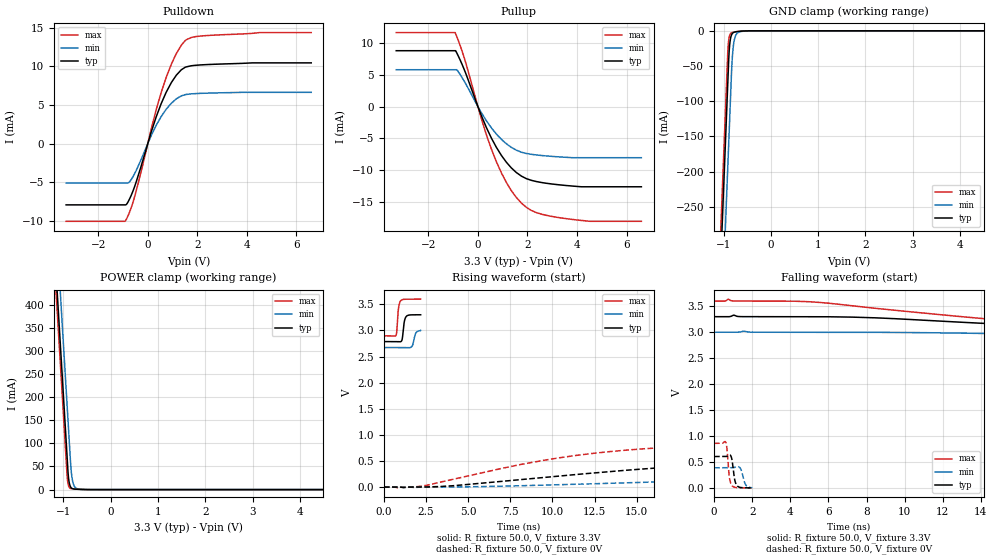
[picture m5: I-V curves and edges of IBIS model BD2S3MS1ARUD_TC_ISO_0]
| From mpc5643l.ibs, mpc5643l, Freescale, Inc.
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| *** New cell (Generated with 5.14beta1 (Sep 20 2010 13:23:23))
[Model]   BD2S3MS1ARUD_TC_ISO_0
Model_type I/O
Polarity   Non-Inverting
Enable   Active-Low
| CAP_THRESHOLD on pad pad is "CMOS" :
| Rising=10.0% of VDDE1   Falling=90.0% of VDDE1
| C_comp min and max val. don't necessarily correlate with the min and max pvt
| but are the smallest and greatest pad capacitance found.
| var   typ   min   max
C_comp   1.37510pF  1.31599pF  1.44239pF
Vinl = 1.05V | Dummy value overriden by next lines
Vinh = 2.34V | Dummy value overriden by next lines
Vmeas = 1.65V   | Reference voltage for timing measurements
Cref  = 25.0pF   | Timing specification test load capacitance value
Rref  = 1.0MOhm   | Timing specification test load resistance value
Vref  = 1.65V   | Timing specification test load voltage
[Model Spec]
| TIME_THRESHOLD on pin ipp_ind is "CORE" :
| Rising=40.0% of VDD   Falling=60.0% of VDD
Vinl 1.30950V 1.19650V 1.40650V
Vinh 1.89650V 1.72150V 2.04550V
| variable   typ   min   max
[Temperature Range] 25.0 150.0 -40.0
| variable   typ   min   max
[Voltage Range] 3.3V 3.0V 3.6V
| variable   typ   min   max
[POWER Clamp Reference] 3.3V 3.0V 3.6V
| variable   typ   min   max
[GND Clamp Reference] 0V 0V 0V
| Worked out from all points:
|   slope of the pulldown table from 0 to 0.495 V, typ, clamps not added: 104 ohm
|   slope of the pullup table from 0 to 0.495 V, typ, clamps not added: 108 ohm
|   GND clamp passes 1 mA (typ) near -0.70 V on its own axis
|   POWER clamp passes 1 mA (typ) near -0.74 V on its own axis
|   rising waveform, R_fixture 50.0, V_fixture 3.3V: 20-80 % time 118ps typ, 147ps min, 106ps max; typ from 2.79 V to 3.3 V
|   falling waveform, R_fixture 50.0, V_fixture 3.3V: 20-80 % time 19.3ns typ, 30.4ns min, 13.8ns max; typ from 3.3 V to 2.79 V
|   rising waveform, R_fixture 50.0, V_fixture 0V: 20-80 % time 15.6ns typ, 31ns min, 9.23ns max; typ from 0 V to 0.604 V
|   falling waveform, R_fixture 50.0, V_fixture 0V: 20-80 % time 141ps typ, 178ps min, 125ps max; typ from 0.604 V to 0 V
[POWER Clamp]
-3.3V     4.118A     4.23A      4.076A
-1.21V    564.8mA    676.6mA    523.5mA
-1.14V    445.8mA    557.6mA    404.5mA
-1.07V    326.8mA    438.6mA    285.5mA
-1V       207.8mA    319.6mA    166.5mA
-920mV    71.78mA    183.6mA    30.49mA
-890mV    26.12mA    132.6mA    8.48mA
-850mV    6.633mA    64.57mA    2.709mA
-820mV    2.915mA    28.96mA    1.809mA
-790mV    1.645mA    13.25mA    1.441mA
-640mV    470.3uA    702.5uA    525.7uA
6.6V      0A         0A         0A
[GND Clamp]
-3.3V     -4.137A    -4.256A    -4.092A
-1.08V    -363mA     -482.1mA   -318.4mA
-920mV    -90.99mA   -210.1mA   -46.4mA
-910mV    -73.99mA   -193.1mA   -29.43mA
-900mV    -56.99mA   -176.1mA   -19.05mA
-880mV    -27.88mA   -142.1mA   -8.77mA
-860mV    -14.01mA   -108.1mA   -4.807mA
-820mV    -4.428mA   -43.91mA   -2.446mA
-790mV    -2.452mA   -20.26mA   -1.874mA
-750mV    -1.501mA   -7.681mA   -1.395mA
-580mV    -299.9uA   -576.1uA   -211.9uA
6.6V      3.169nA    967.5nA    21.29pA
| variable   typ   min   max
[Pullup Reference] 3.3V 3.0V 3.6V
| variable   typ   min   max
[Pulldown Reference] 0V 0V 0V
[Pullup]
-3.3V     8.847mA    5.839mA    11.72mA
-920mV    8.847mA    5.839mA    11.72mA
-850mV    8.461mA    5.839mA    11.04mA
-530mV    5.641mA    3.871mA    7.427mA
340mV     -3.289mA   -2.224mA   -4.425mA
740mV     -6.399mA   -4.306mA   -8.659mA
950mV     -7.722mA   -5.179mA   -10.49mA
1.35V     -9.688mA   -6.439mA   -13.28mA
1.96V     -11.39mA   -7.41mA    -15.93mA
2.57V     -12mA      -7.725mA   -17mA
3.78V     -12.54mA   -8.06mA    -17.82mA
6.6V      -12.67mA   -8.071mA   -18.13mA
[Pulldown]
-3.3V     -7.939mA   -5.109mA   -10.07mA
-900mV    -7.939mA   -5.109mA   -9.995mA
-750mV    -7.258mA   -4.993mA   -8.98mA
-540mV    -5.638mA   -3.948mA   -6.973mA
340mV     3.462mA    2.363mA    4.387mA
740mV     6.62mA     4.428mA    8.533mA
1.15V     8.842mA    5.781mA    11.64mA
1.35V     9.537mA    6.164mA    12.71mA
1.55V     9.918mA    6.352mA    13.42mA
1.96V     10.14mA    6.469mA    13.85mA
2.57V     10.25mA    6.538mA    14.01mA
6.6V      10.44mA    6.629mA    14.36mA
[Ramp]
dV/dt_r 362.31485mV/15.58399ns 232.2189mV/30.96259ns 515.12251mV/9.22779ns
dV/dt_f 308.176mV/19.33668ns 196.13161mV/30.38952ns 422.04011mV/13.82957ns
R_load = 50.0
| Removed startup time: 0s 0s 0s  .
| Removed end time: 2.177ns.
[Rising Waveform]
R_fixture   = 50.0
V_fixture   = 3.3V
V_fixture_min = 3.0V
V_fixture_max = 3.6V
0s        2.786V     2.673V     2.897V
720ps     2.786V     2.673V     2.908V
867ps     2.785V     2.673V     3.432V
1.008ns   2.787V     2.673V     3.573V
1.091ns   2.846V     2.673V     3.59V
1.211ns   3.173V     2.673V     3.597V
1.317ns   3.265V     2.673V     3.598V
1.658ns   3.298V     2.69V      3.599V
1.886ns   3.299V     2.945V     3.599V
2.179ns   3.3V       3V         3.6V
| Removed startup time: 0s 0s 0s  .
| Removed end time: 132.1ns.
[Falling Waveform]
R_fixture   = 50.0
V_fixture   = 3.3V
V_fixture_min = 3.0V
V_fixture_max = 3.6V
0s        3.3V       3V         3.6V
750ps     3.299V     3V         3.638V
1.05ns    3.329V     2.999V     3.601V
5.25ns    3.3V       3V         3.582V
9.1ns     3.268V     2.997V     3.438V
19.55ns   3.072V     2.936V     3.101V
29.55ns   2.917V     2.859V     2.952V
40.35ns   2.838V     2.784V     2.918V
58.95ns   2.803V     2.716V     2.902V
132.2ns   2.786V     2.673V     2.897V
| Removed startup time: 0s 0s 0s  .
| Removed end time: 109.6ns.
[Rising Waveform]
R_fixture   = 50.0
V_fixture   = 0V
V_fixture_min = 0V
V_fixture_max = 0V
0s        14.09nV    564.3nV    12.88nV
800ps     202.4uV    608nV      -15.61mV
2.35ns    773.3uV    -178.3uV   23.37mV
8.15ns    142.9mV    25.2mV     434.3mV
12.35ns   266.9mV    61.81mV    643mV
16.5ns    372.1mV    100.6mV    754.9mV
21.4ns    461.4mV    147.5mV    814.9mV
33ns      561.5mV    244.3mV    852mV
51.65ns   597.1mV    332.7mV    857.9mV
109.7ns   603.9mV    387mV      858.5mV
| Removed startup time: 0s 0s 0s  .
| Removed end time: 1.987ns.
[Falling Waveform]
R_fixture   = 50.0
V_fixture   = 0V
V_fixture_min = 0V
V_fixture_max = 0V
0s        603.9mV    387.1mV    858.5mV
614ps     603.6mV    387.1mV    877.5mV
677ps     609.3mV    387.1mV    753.5mV
800ps     633.3mV    386.9mV    213.2mV
942ps     537.4mV    386.8mV    43.15mV
1.074ns   173mV      393.9mV    11.99mV
1.187ns   50.48mV    406.1mV    4.436mV
1.399ns   6.655mV    363.9mV    874.9uV
1.673ns   798.1uV    51.41mV    246.4uV
1.989ns   68.69uV    39.6uV     138.5uV
